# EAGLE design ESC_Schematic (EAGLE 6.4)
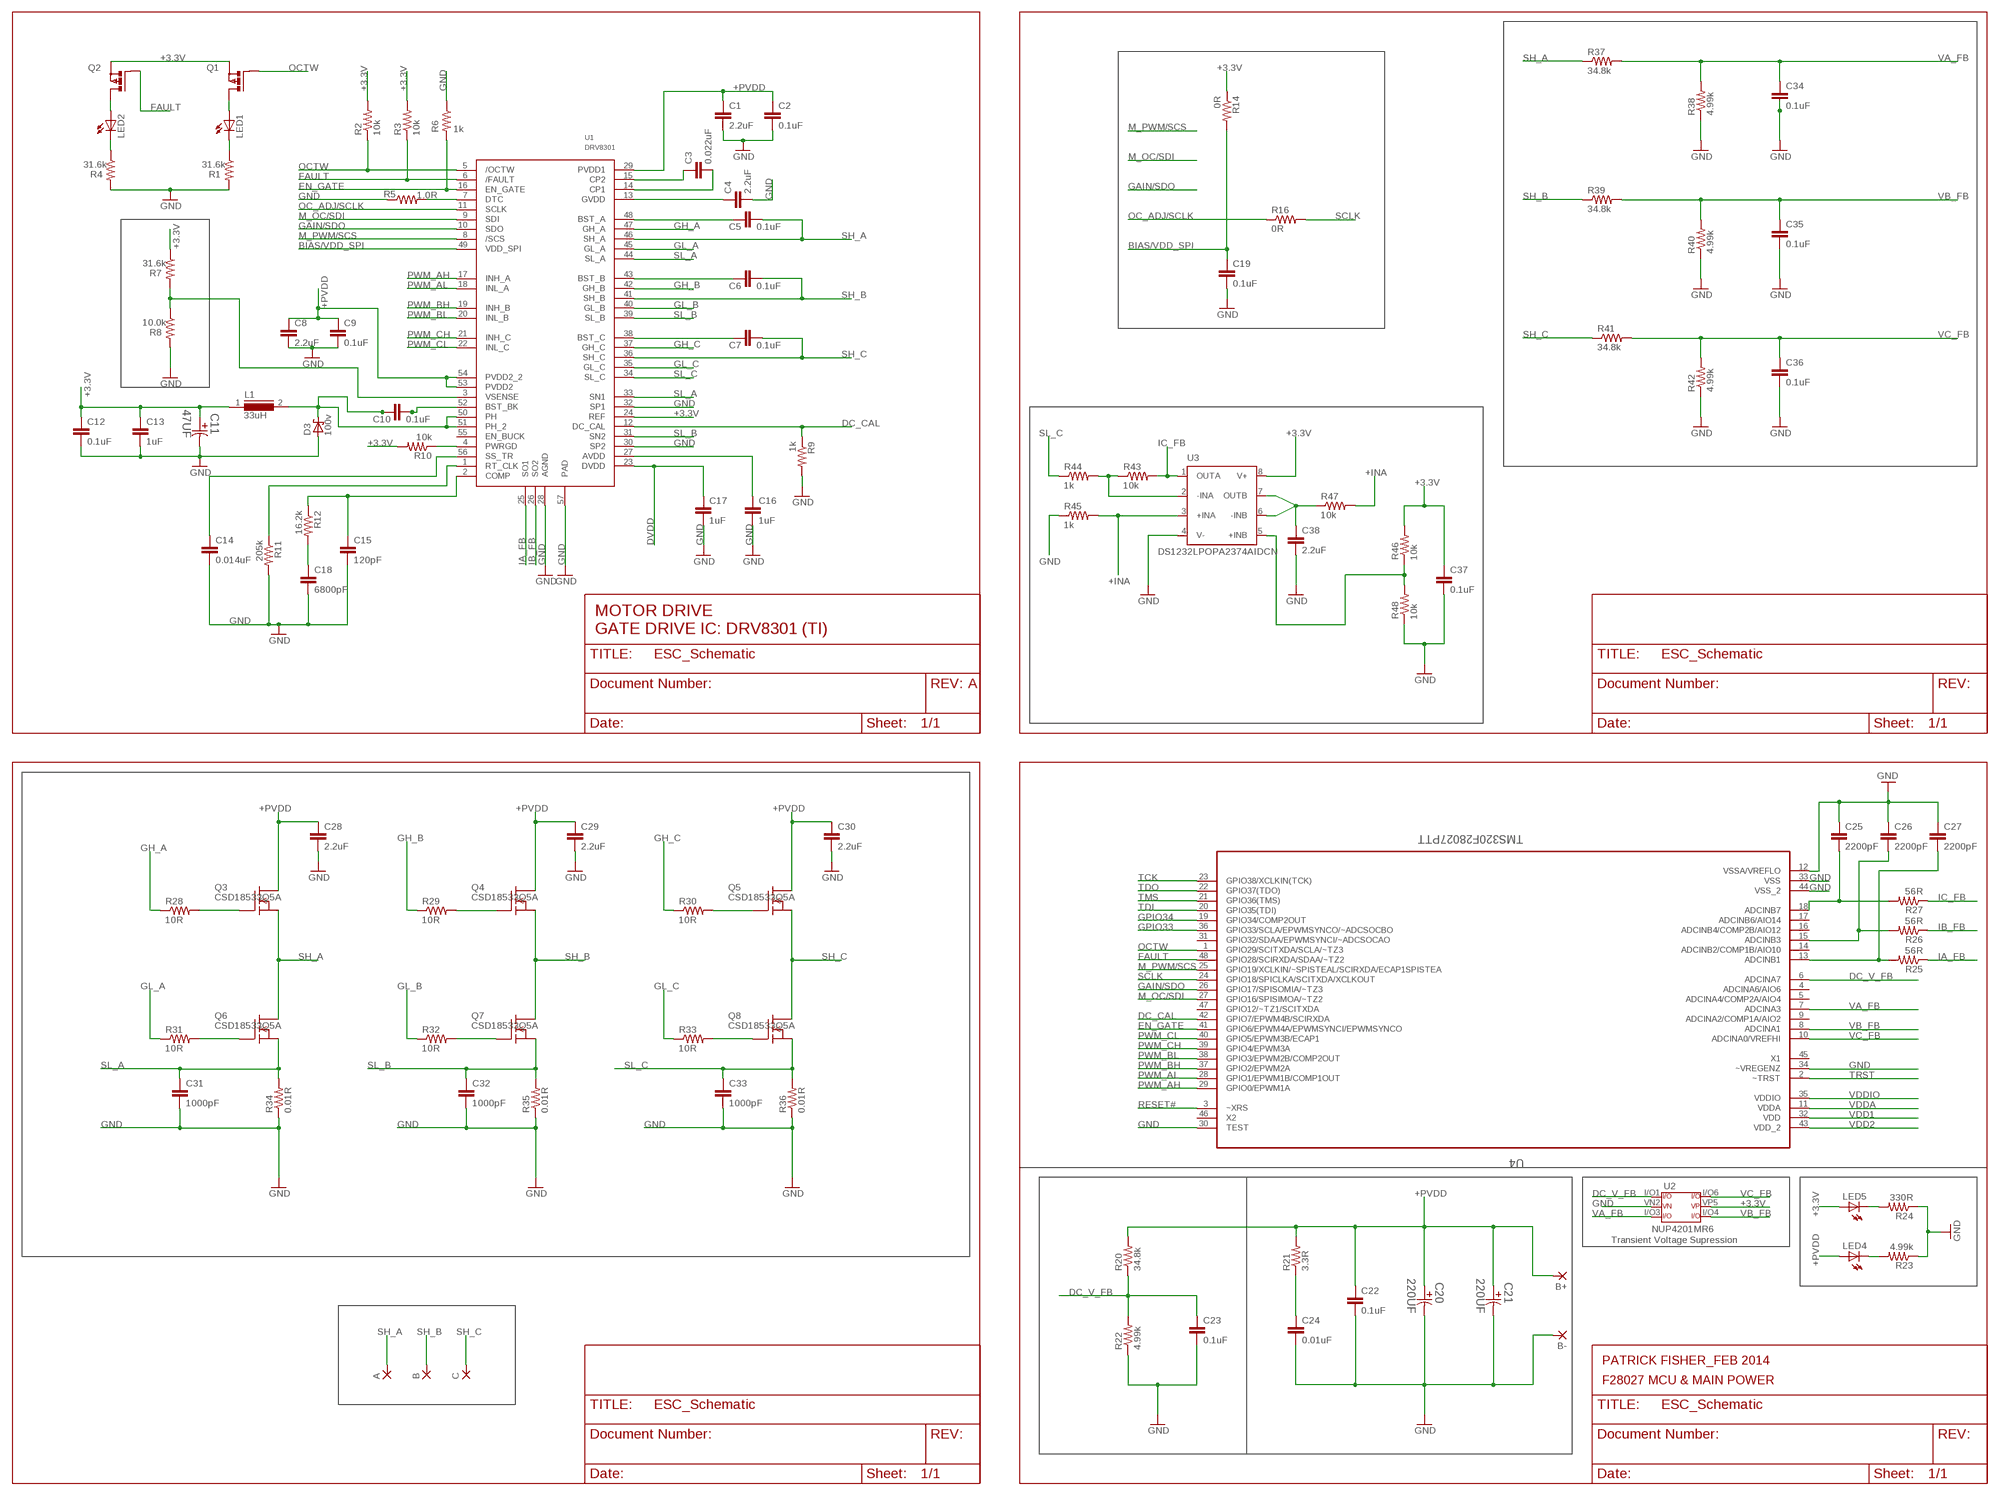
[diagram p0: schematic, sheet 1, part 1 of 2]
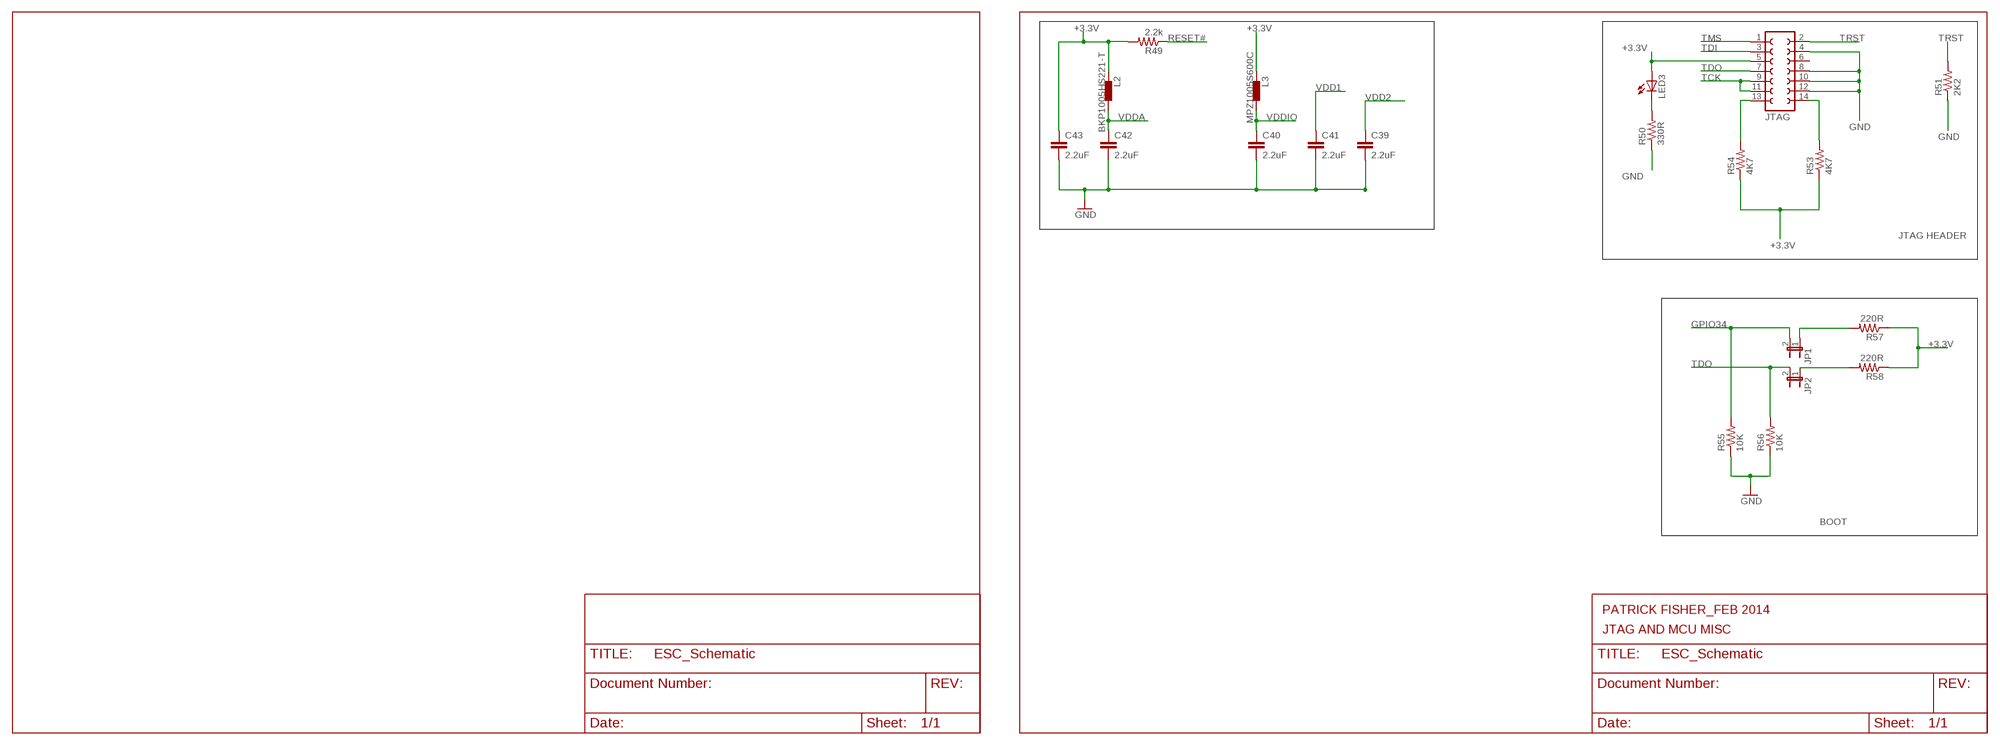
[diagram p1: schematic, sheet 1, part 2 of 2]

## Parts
A  WIREPAD4,16O1,6  [4,16O1,6]
B  WIREPAD4,16O1,6  [4,16O1,6]
B+  WIREPAD4,16O1,6  [4,16O1,6]
B-  WIREPAD4,16O1,6  [4,16O1,6]
C  WIREPAD4,16O1,6  [4,16O1,6]
C1  2.2uF  C-EUC1210  [C1210]
C2  0.1uF  C-EUC0603  [C0603]
C3  0.022uF  C-EUC0603  [C0603]
C4  2.2uF  C-EUC0805  [C0805]
C5  0.1uF  C-EUC0603  [C0603]
C6  0.1uF  C-EUC0603  [C0603]
C7  0.1uF  C-EUC0603  [C0603]
C8  2.2uF  C-EUC1210  [C1210]
C9  0.1uF  C-EUC0603  [C0603]
C10  0.1uF  C-EUC0603  [C0603]
C11  47UF  EEE-FK1E470P-CASE-D  [CAPAE660X610N]
C12  0.1uF  C-EUC0603  [C0603]
C13  1uF  C-EUC0603  [C0603]
C14  0.014uF  C-EUC0603  [C0603]
C15  120pF  C-EUC0603  [C0603]
C16  1uF  C-EUC0603  [C0603]
C17  1uF  C-EUC0603  [C0603]
C18  6800pF  C-EUC0603  [C0603]
C19  0.1uF  C-EUC0603  [C0603]
C20  220UF  EEE-FC1H221P-CASE-G  [CAPAE1030X1050N]
C21  220UF  EEE-FC1H221P-CASE-G  [CAPAE1030X1050N]
C22  0.1uF  C-EUC0603  [C0603]
C23  0.1uF  C-EUC0603  [C0603]
C24  0.01uF  C-EUC0603  [C0603]
C25  2200pF  C-EUC0603  [C0603]
C26  2200pF  C-EUC0603  [C0603]
C27  2200pF  C-EUC0603  [C0603]
C28  2.2uF  C-EUC1210  [C1210]
C29  2.2uF  C-EUC1210  [C1210]
C30  2.2uF  C-EUC1210  [C1210]
C31  1000pF  C-EUC0603  [C0603]
C32  1000pF  C-EUC0603  [C0603]
C33  1000pF  C-EUC0603  [C0603]
C34  0.1uF  C-EUC0603  [C0603]
C35  0.1uF  C-EUC0603  [C0603]
C36  0.1uF  C-EUC0603  [C0603]
C37  0.1uF  C-EUC0603  [C0603]
C38  2.2uF  C-EUC0603  [C0603]
C39  2.2uF  C-EUC0402K  [C0402K]
C40  2.2uF  C-EUC0402K  [C0402K]
C41  2.2uF  C-EUC0402K  [C0402K]
C42  2.2uF  C-EUC0402K  [C0402K]
C43  2.2uF  C-EUC0402K  [C0402K]
D3  100v  SCHOTTKY-DIODESMD  [SMB]
JP1  JP1E  [JP1]
JP2  JP1E  [JP1]
JTAG  FE07-2  [FE07-2]
L1  33uH  DR74  [DR74]
L2  220R  BLM15HB121SN1  [0402]
L3  60R  BLM15HB121SN1  [0402]
LED1  LEDCHIP-LED0805  [CHIP-LED0805]
LED2  LEDCHIP-LED0805  [CHIP-LED0805]
LED3  LEDCHIP-LED0805  [CHIP-LED0805]
LED4  LEDCHIP-LED0805  [CHIP-LED0805]
LED5  LEDCHIP-LED0805  [CHIP-LED0805]
Q1  P-MOSFET-SO8  [SOT23]
Q2  P-MOSFET-SO8  [SOT23]
Q3  CSD18533Q5A  [SON5*6]
Q4  CSD18533Q5A  [SON5*6]
Q5  CSD18533Q5A  [SON5*6]
Q6  CSD18533Q5A  [SON5*6]
Q7  CSD18533Q5A  [SON5*6]
Q8  CSD18533Q5A  [SON5*6]
R1  31.6k  R-US_R0603  [R0603]
R2  10k  R-US_R0603  [R0603]
R3  10k  R-US_R0603  [R0603]
R4  31.6k  R-US_R0603  [R0603]
R5  1.0R  R-US_R0603  [R0603]
R6  1k  R-US_R0603  [R0603]
R7  31.6k  R-US_R0603  [R0603]
R8  10.0k  R-US_R0603  [R0603]
R9  1k  R-US_R0603  [R0603]
R10  10k  R-US_R0603  [R0603]
R11  205k  R-US_R0603  [R0603]
R12  16.2k  R-US_R0603  [R0603]
R14  0R  R-US_R0603  [R0603]
R16  0R  R-US_R0603  [R0603]
R20  34.8k  R-US_R0603  [R0603]
R21  3.3R  R-US_R1206  [R1206]
R22  4.99k  R-US_R0603  [R0603]
R23  4.99k  R-US_R0603  [R0603]
R24  330R  R-US_R0603  [R0603]
R25  56R  R-US_R0603  [R0603]
R26  56R  R-US_R0603  [R0603]
R27  56R  R-US_R0603  [R0603]
R28  10R  R-US_R0603  [R0603]
R29  10R  R-US_R0603  [R0603]
R30  10R  R-US_R0603  [R0603]
R31  10R  R-US_R0603  [R0603]
R32  10R  R-US_R0603  [R0603]
R33  10R  R-US_R0603  [R0603]
R34  0.01R  R-US_R2512  [R2512]
R35  0.01R  R-US_R2512  [R2512]
R36  0.01R  R-US_R2512  [R2512]
R37  34.8k  R-US_R0603  [R0603]
R38  4.99k  R-US_R0603  [R0603]
R39  34.8k  R-US_R0603  [R0603]
R40  4.99k  R-US_R0603  [R0603]
R41  34.8k  R-US_R0603  [R0603]
R42  4.99k  R-US_R0603  [R0603]
R43  10k  R-US_R0603  [R0603]
R44  1k  R-US_R0603  [R0603]
R45  1k  R-US_R0603  [R0603]
R46  10k  R-US_R0603  [R0603]
R47  10k  R-US_R0603  [R0603]
R48  10k  R-US_R0603  [R0603]
R49  2.2k  R-US_R0402  [R0402]
R50  330R  R-US_R0603  [R0603]
R51  2K2  R-US_R0603  [R0603]
R53  4K7  R-US_R0603  [R0603]
R54  4K7  R-US_R0603  [R0603]
R55  10K  R-US_R0603  [R0603]
R56  10K  R-US_R0603  [R0603]
R57  220R  R-US_R0603  [R0603]
R58  220R  R-US_R0603  [R0603]
U1  DRV8301  [TSSOP56P]
U2  DIL6  [SOT23-6]
U3  DS1232LPOPA2374AIDCN  [DCN-R-PDSO-G8]
U4  TMS320F28027PTT  [QFP50P900X900X160-48N]

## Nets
+3.3V: C11.1 C12.1 C13.1 C37.1 C43.1 JTAG.5 L1.1 L2.1 L3.1 LED3.A LED5.A Q1.2(S) Q2.2(S) R2.2 R3.2 R7.1 R10.2 R14.1 R46.2 R49.2 R53.1 R54.1 R57.1 R58.1 U1.24(REF) U2.VP5 U3.8(V+)
+INA: R45.2 R47.2 U3.3(+INA)
+PVDD: B+.1(P) C1.1 C2.1 C8.1 C9.1 C20.1 C21.1 C22.1 C28.1 C29.1 C30.1 LED4.A Q3.5(D) Q3.6(D) Q3.7(D) Q3.8(D) Q3.9(D) Q4.5(D) Q4.6(D) Q4.7(D) Q4.8(D) Q4.9(D) Q5.5(D) Q5.6(D) Q5.7(D) Q5.8(D) Q5.9(D) R20.2 R21.2 U1.29(PVDD1) U1.53(PVDD2) U1.54(PVDD2_2)
BIAS/VDD_SPI: C19.1 R14.2 U1.49(VDD_SPI)
DC_CAL: R9.1 U1.12(DC_CAL) U4.42(GPIO7/EPWM4B/SCIRXDA)
DC_V_FB: C23.1 R20.1 R22.2 U2.I/O1 U4.6(ADCINA7)
DVDD: C17.1 U1.23(DVDD)
EN_GATE: R6.2 U1.16(EN_GATE) U4.41(GPIO6/EPWM4A/EPWMSYNCI/EPWMSYNCO)
FAULT: Q2.1(G) R3.1 U1.6(/FAULT) U4.48(GPIO28/SCIRXDA/SDAA/~TZ2)
GAIN/SDO: U1.10(SDO) U4.26(GPIO17/SPISOMIA/~TZ3)
GH_A: R28.1 U1.47(GH_A)
GH_B: R29.1 U1.42(GH_B)
GH_C: R30.1 U1.37(GH_C)
GL_A: R31.1 U1.45(GL_A)
GL_B: R32.1 U1.40(GL_B)
GL_C: R33.1 U1.35(GL_C)
GND: B-.1(P) C1.2 C2.2 C4.2 C8.2 C9.2 C11.2 C12.2 C13.2 C14.2 C15.2 C16.2 C17.2 C18.2 C19.2 C20.2 C21.2 C22.2 C23.2 C24.2 C25.1 C26.1 C27.1 C28.2 C29.2 C30.2 C31.2 C32.2 C33.2 C34.2 C35.2 C36.2 C37.2 C38.2 C39.2 C40.2 C41.2 C42.2 C43.2 D3.A JTAG.4 JTAG.8 JTAG.10 JTAG.12 R1.2 R4.2 R5.1 R6.1 R8.2 R9.2 R11.2 R22.1 R23.1 R24.1 R34.1 R35.1 R36.1 R38.1 R40.1 R42.1 R45.1 R48.1 R50.1 R51.1 R55.1 R56.1 U1.28(AGND) U1.30(SP2) U1.32(SP1) U1.57(PAD) U2.VN2 U3.4(V-) U4.12(VSSA/VREFLO) U4.30(TEST) U4.33(VSS) U4.34(~VREGENZ) U4.44(VSS_2)
GPIO33: U4.36(GPIO33/SCLA/EPWMSYNCO/~ADCSOCBO)
GPIO34: JP1.2 R55.2 U4.19(GPIO34/COMP2OUT)
IA_FB: R25.1 U1.25(SO1)
IB_FB: R26.1 U1.26(SO2)
IC_FB: R27.1 R43.2 U3.1(OUTA)
M_OC/SDI: U1.9(SDI) U4.27(GPIO16/SPISIMOA/~TZ2)
M_PWM/SCS: U1.8(/SCS) U4.25(GPIO19/XCLKIN/~SPISTEAL/SCIRXDA/ECAP1SPISTEA)
N$1: R10.1 U1.4(PWRGD)
N$2: R7.2 R8.1 U1.3(VSENSE)
N$3: C10.2 U1.52(BST_BK)
N$4: R5.2 U1.7(DTC)
N$5: C10.1 D3.C L1.2 U1.50(PH) U1.51(PH_2)
N$6: C18.1 R12.2
N$7: C14.1 U1.56(SS_TR)
N$8: LED1.A Q1.3(D)
N$9: C15.1 R12.1 U1.2(COMP)
N$10: C3.1 U1.15(CP2)
N$11: R11.1 U1.1(RT_CLK)
N$12: C3.2 U1.14(CP1)
N$13: C4.1 U1.13(GVDD)
N$14: C6.1 U1.43(BST_B)
N$15: C5.1 U1.48(BST_A)
N$16: C7.1 U1.38(BST_C)
N$17: LED1.C R1.1
N$18: LED2.A Q2.3(D)
N$19: LED2.C R4.1
N$21: C38.1 R47.1 U3.6(-INB) U3.7(OUTB)
N$22: R46.1 R48.2 U3.5(+INB)
N$23: C16.1 U1.27(AVDD)
N$24: Q3.4(G) R28.2
N$25: Q4.4(G) R29.2
N$26: R43.1 R44.2 U3.2(-INA)
N$27: Q5.4(G) R30.2
N$28: Q7.4(G) R32.2
N$29: Q8.4(G) R33.2
N$30: Q6.4(G) R31.2
N$31: C26.2 R26.2 U4.15(ADCINB3)
N$32: C27.2 R25.2 U4.13(ADCINB1)
N$33: LED3.C R50.2
N$34: LED4.C R23.2
N$35: C25.2 R27.2 U4.18(ADCINB7)
N$36: LED5.C R24.2
N$39: JTAG.13 R54.2
N$40: JTAG.14 R53.2
N$42: JP1.1 R57.2
N$44: C24.1 R21.1
N$45: JP2.1 R58.2
OC_ADJ/SCLK: R16.1 U1.11(SCLK)
OCTW: Q1.1(G) R2.1 U1.5(/OCTW) U4.1(GPIO29/SCITXDA/SCLA/~TZ3)
PWM_AH: U1.17(INH_A) U4.29(GPIO0/EPWM1A)
PWM_AL: U1.18(INL_A) U4.28(GPIO1/EPWM1B/COMP1OUT)
PWM_BH: U1.19(INH_B) U4.37(GPIO2/EPWM2A)
PWM_BL: U1.20(INL_B) U4.38(GPIO3/EPWM2B/COMP2OUT)
PWM_CH: U1.21(INH_C) U4.39(GPIO4/EPWM3A)
PWM_CL: U1.22(INL_C) U4.40(GPIO5/EPWM3B/ECAP1)
RESET#: R49.1 U4.3(~XRS)
SCLK: R16.2 U4.24(GPIO18/SPICLKA/SCITXDA/XCLKOUT)
SH_A: A.1(P) C5.2 Q3.1(S) Q3.2(S) Q3.3(S) Q6.5(D) Q6.6(D) Q6.7(D) Q6.8(D) Q6.9(D) R37.1 U1.46(SH_A)
SH_B: B.1(P) C6.2 Q4.1(S) Q4.2(S) Q4.3(S) Q7.5(D) Q7.6(D) Q7.7(D) Q7.8(D) Q7.9(D) R39.1 U1.41(SH_B)
SH_C: C7.2 C.1(P) Q5.1(S) Q5.2(S) Q5.3(S) Q8.5(D) Q8.6(D) Q8.7(D) Q8.8(D) Q8.9(D) R41.1 U1.36(SH_C)
SL_A: C31.1 Q6.1(S) Q6.2(S) Q6.3(S) R34.2 U1.33(SN1) U1.44(SL_A)
SL_B: C32.1 Q7.1(S) Q7.2(S) Q7.3(S) R35.2 U1.31(SN2) U1.39(SL_B)
SL_C: C33.1 Q8.1(S) Q8.2(S) Q8.3(S) R36.2 R44.1 U1.34(SL_C)
TCK: JTAG.9 JTAG.11 U4.23(GPIO38/XCLKIN(TCK))
TDI: JTAG.3 U4.20(GPIO35(TDI))
TDO: JP2.2 JTAG.7 R56.2 U4.22(GPIO37(TDO))
TMS: JTAG.1 U4.21(GPIO36(TMS))
TRST: JTAG.2 R51.2 U4.2(~TRST)
VA_FB: C34.1 R37.2 R38.2 U2.I/O3 U4.7(ADCINA3)
VB_FB: C35.1 R39.2 R40.2 U2.I/O4 U4.8(ADCINA1)
VC_FB: C36.1 R41.2 R42.2 U2.I/O6 U4.10(ADCINA0/VREFHI)
VDD1: C41.1 U4.32(VDD)
VDD2: C39.1 U4.43(VDD_2)
VDDA: C42.1 L2.2 U4.11(VDDA)
VDDIO: C40.1 L3.2 U4.35(VDDIO)
Unconnected: JTAG.6 U1.55(EN_BUCK) U4.4(ADCINA6/AIO6) U4.5(ADCINA4/COMP2A/AIO4) U4.9(ADCINA2/COMP1A/AIO2) U4.14(ADCINB2/COMP1B/AIO10) U4.16(ADCINB4/COMP2B/AIO12) U4.17(ADCINB6/AIO14) U4.31(GPIO32/SDAA/EPWMSYNCI/~ADCSOCAO) U4.45(X1) U4.46(X2) U4.47(GPIO12/~TZ1/SCITXDA)

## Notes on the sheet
- MOTOR DRIVE
  GATE DRIVE IC: DRV8301 (TI)
- A
- NUP4201MR6
- Transient Voltage Supression
- PATRICK FISHER_FEB 2014
- F28027 MCU & MAIN POWER
- BKP1005HS221-T | MPZ1005S600C
- JTAG HEADER
- BOOT
- PATRICK FISHER_FEB 2014
- JTAG AND MCU MISC

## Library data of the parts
A B B+ B- C = wirepad:WIREPAD: Wire PAD connect wire on PCB
C1-C10 C12-C19 C22-C43 = rcl:C-EU: CAPACITOR, European symbol
C11 = Panasonic-EEEFK_EEEFP:EEE-: Aluminum Electrolytic Capacitors,Surface Mount Type; MPN: EEE-FK1E470P; OC_FARNELL: 9695753; OC_NEWARK: 87K0936; PACKAGE: CASE-D; SUPPLIER: PANASONIC; TOLERANCE: ±20 %; VOLTAGERATING: 25V
C20 C21 = Panasonic-EEE0_EEE1_EEE2_EEEFC:EEE-: Aluminum Electrolytic Capacitors,Surface Mount Type; MPN: EEE-FC1H221P; OC_FARNELL: 2284641; OC_NEWARK: 53W3650; PACKAGE: CASE-G; SUPPLIER: PANASONIC; TOLERANCE: 20%; VOLTAGERATING: 50V
D3 = diode:SCHOTTKY-DIODE: Schottky Diode
JP1 JP2 = jumper:JP1E: JUMPER
JTAG = con-lsta:FE07-2: FEMALE HEADER; OC_FARNELL: unknown; OC_NEWARK: unknown
L1 = inductors:DR74: High Power Density, High Efficiency, Shielded Inductors
L2 L3 = inductors:BLM15H: EMIFIL (R) Chip Ferrite Bead for GHz Noise
LED1-LED5 = led:LED: LED
Q1 Q2 = FET SOT23(good):P-MOSFET-SO8: P-Channel MOSFET Example: FDS4435A; P-Channel Logic Level PowerTrench® MOSFET FDS4465; P-Channel 1.8V Specified PowerTrench® MOSFET Source: www.fairchildsemi.com
Q3-Q8 = CSD18533Q5A:CSD18533Q5A: 60V N-Channel PowerTrench TM MOSFET FAIRCHILD FDS5680.pdf
R1-R12 R14 R16 R20-R51 R53-R58 = resistor:R-US_: RESISTOR, American symbol
U1 = sc_usercreated:DRV8301
U2 = NUP4201MR6:DIL6: Dual In Line / Socket
U3 = OPA2374AIDCN:DS1232LP: Low Power MicroMonitor Chip Source: DALLAS SEMICONDUCTOR .. 1232lp.pdf
U4 = F28027F:TMS320F28027PTT: Piccolo Microcontrollers; MPN: TMS320F28027PTT; OC_FARNELL: 2113746; OC_NEWARK: 50R8075; PACKAGE: PQFP-48; SUPPLIER: Texas Instruments

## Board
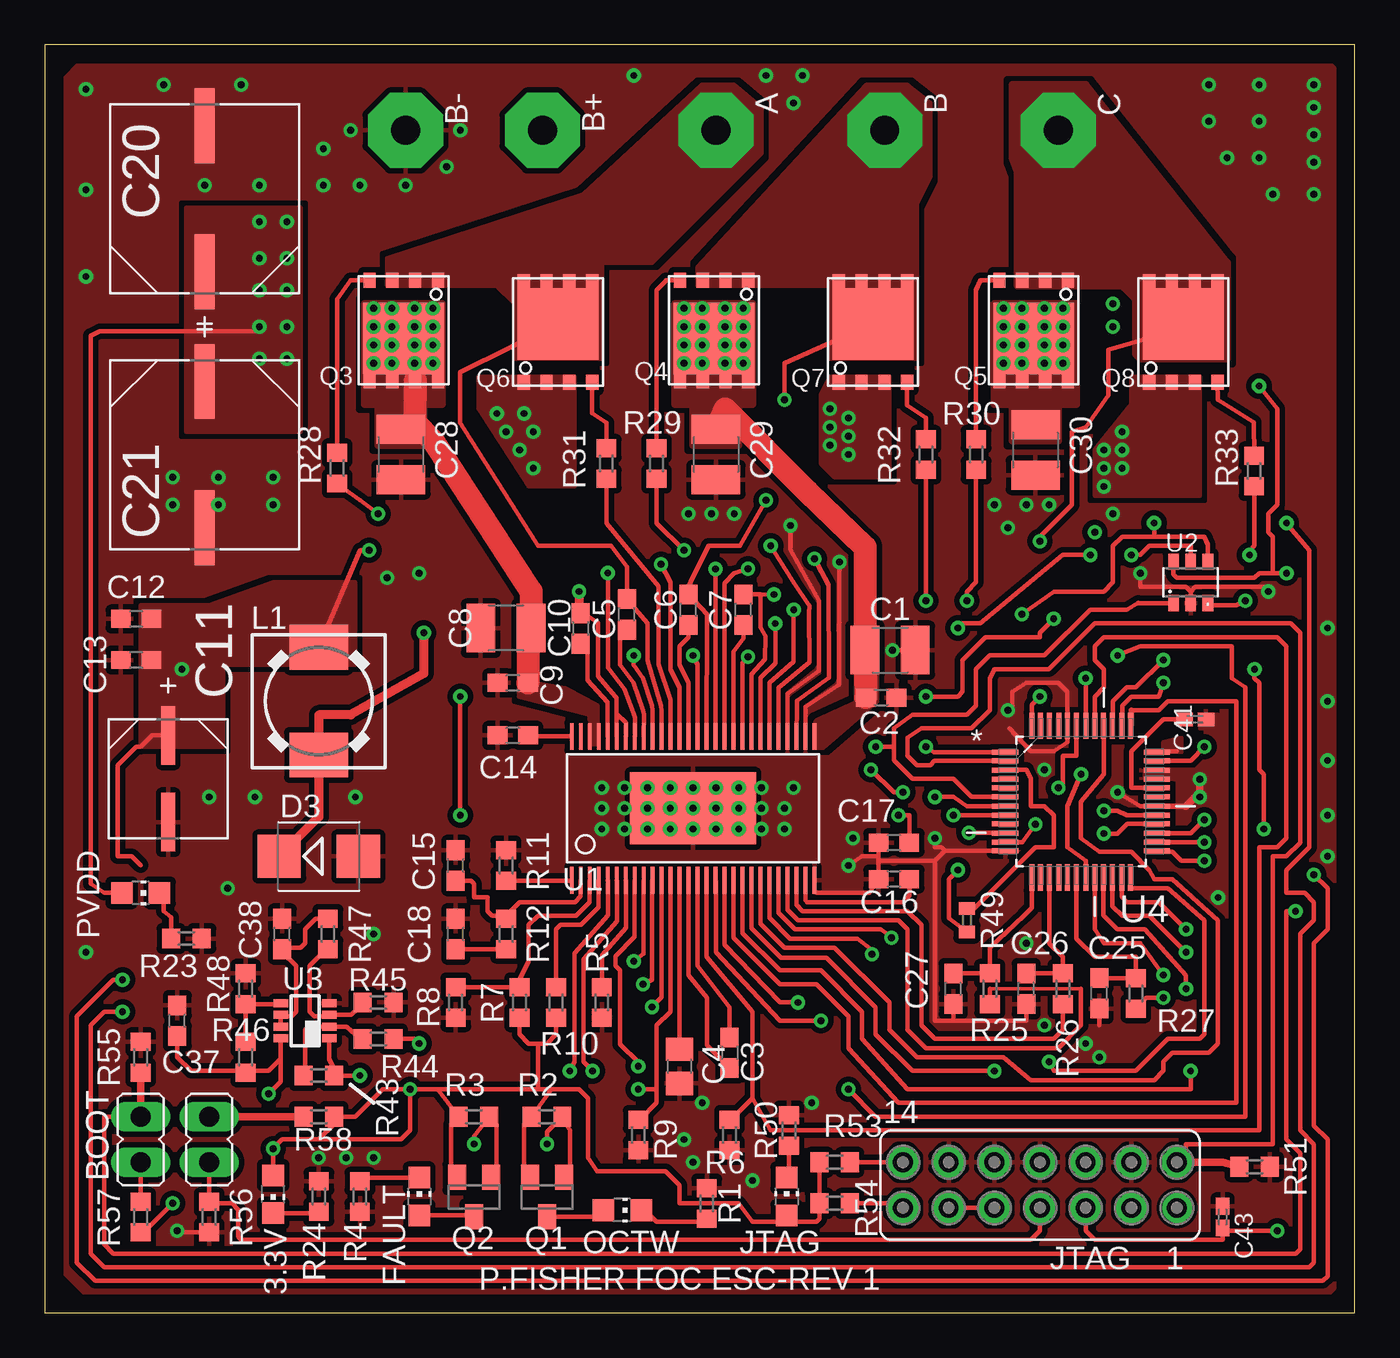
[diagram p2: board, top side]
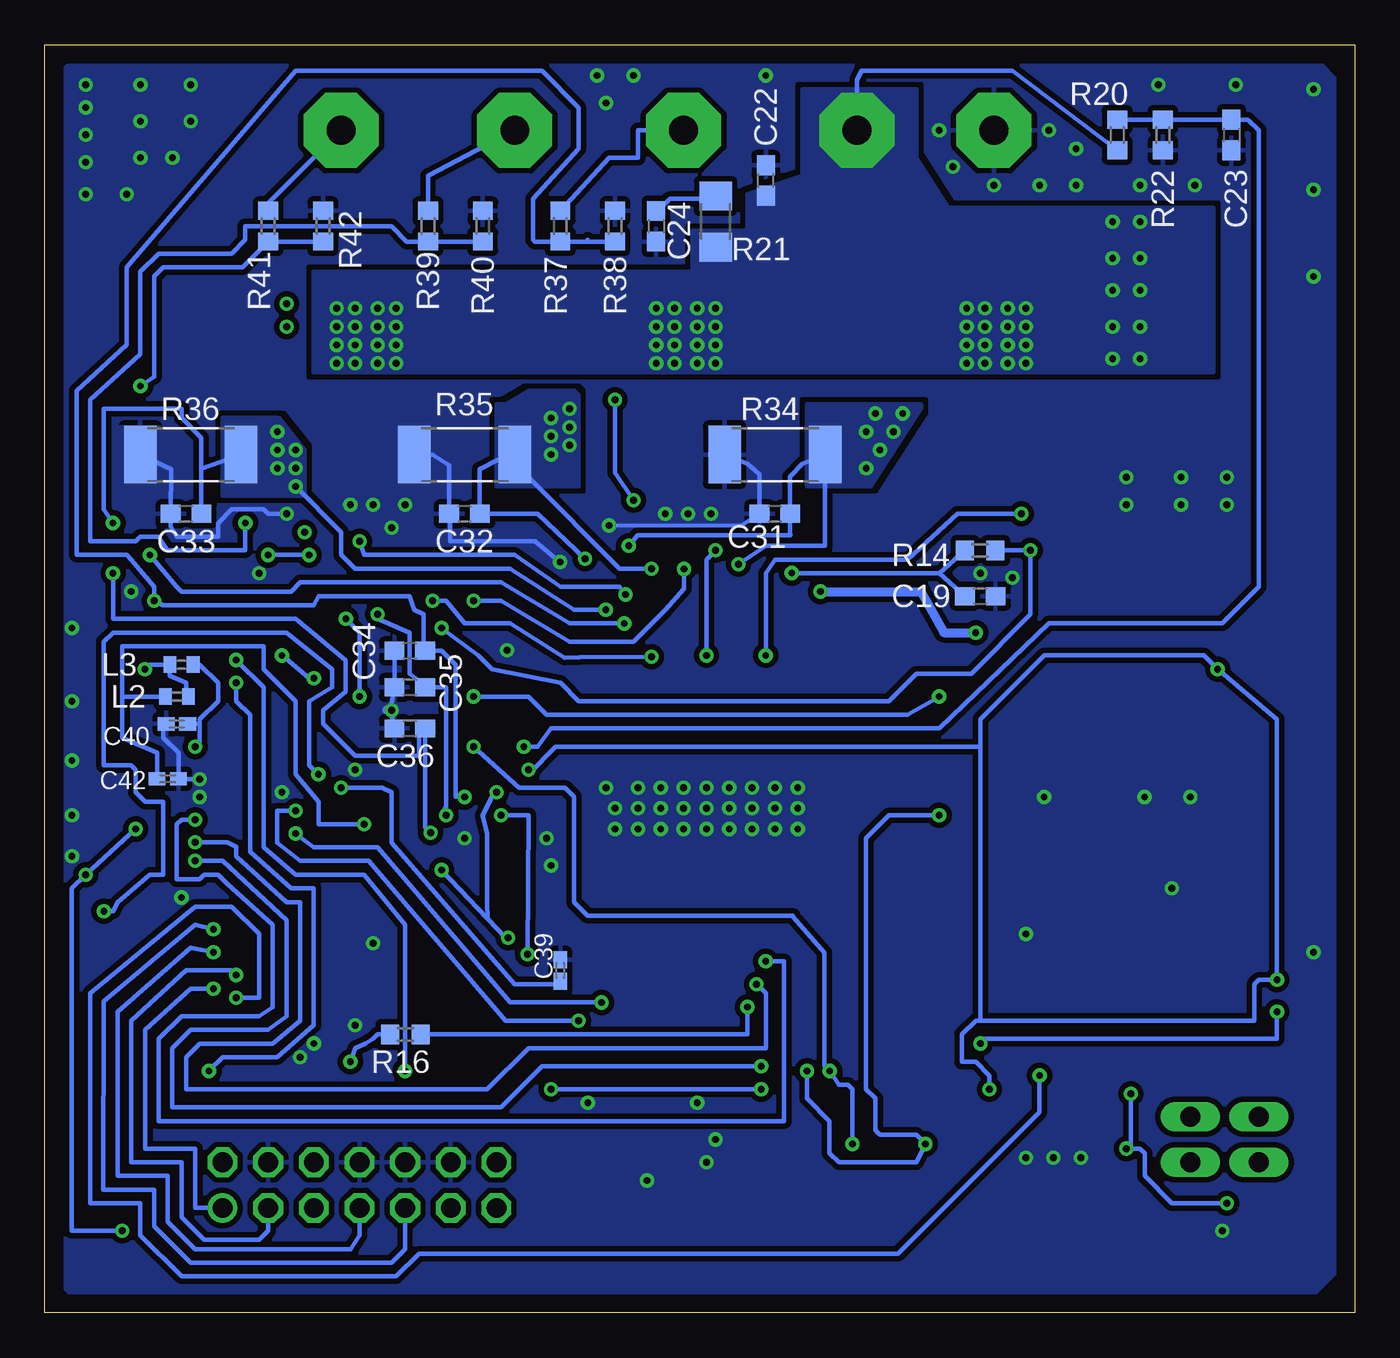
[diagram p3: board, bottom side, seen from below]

Size 72.88 x 70.54 mm. Coordinates in mm from the lower left corner, seen from the top.
Outline: 0,0 72.88,0 72.88,70.54 0,70.54 0,0
Copper layers (1*16): Top 0.035mm / dielectric 1.5mm / Bottom 0.035mm
Design rules "default *": minimum track width 5mil, minimum drill 15mil, track to track 8mil, track to pad 6mil, pad to pad 6mil, via to via 10mil, smd to smd 6mil, copper to edge 40mil, drill to drill 8mil, minimum pad ring 10mil, minimum via ring 8mil, stop-mask expansion 4mil, vias tented up to drill 0mil, thermal gap 12mil

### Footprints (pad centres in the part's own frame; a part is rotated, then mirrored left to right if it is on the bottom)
4,16O1,6 = drill 1.6 pad 4.166 octagon: 1 0,0
C1210 = smd 1.6 x 2.7: 1 -1.4,0; 2 1.4,0
C0603 = smd 1.1 x 1: 1 -0.85,0; 2 0.85,0
C0805 = smd 1.3 x 1.5: 1 -0.95,0; 2 0.95,0
CAPAE660X610N = smd 3.251 x 0.762: 1 -2.413,0; 2 2.413,0
CAPAE1030X1050N = smd 4.166 x 1.092: 1 -4.064,0; 2 4.064,0
C0402K = smd 0.925 x 0.74: 1 -0.6,0; 2 0.6,0
SMB = smd 2.4 x 2.4: A 2.2,0; C -2.2,0
JP1 = drill 1.1 long: 1 0,-1.27; 2 0,1.27
FE07-2 = drill 1.1: 1 -7.62,1.27 | drill 1.1 octagon: 2 -7.62,-1.27; 3 -5.08,1.27; 4 -5.08,-1.27; 5 -2.54,1.27; 6 -2.54,-1.27; 7 0,1.27; 8 0,-1.27; 9 2.54,1.27; 10 2.54,-1.27; 11 5.08,1.27; 12 5.08,-1.27; 13 7.62,1.27; 14 7.62,-1.27
DR74 = smd 2.5 x 3.25: 1 -3,0; 2 3,0
0402 = smd 0.7 x 0.9: 1 -0.65,0; 2 0.65,0
CHIP-LED0805 = smd 1.2 x 1.2: A 0,-1.05; C 0,1.05
SOT23 = smd 1 x 1.4: 1 -0.95,-1.2; 2 0.95,-1.2; 3 0,1
SON5*6 = smd 0.85 x 0.68: 1 -3.095,1.805; 2 -3.095,0.535; 3 -3.095,-0.735; 4 -3.095,-2.005; 5 2.495,-2.005; 6 2.495,-0.735; 7 2.495,0.535; 8 2.495,1.805 | smd 4 x 4.5: 9 0.15,-0.1
R0603 = smd 1 x 1.1: 1 -0.85,0; 2 0.85,0
R1206 = smd 1.6 x 1.803: 1 -1.422,0; 2 1.422,0
R2512 = smd 1.8 x 3.2: 1 -2.8,0; 2 2.8,0
R0402 = smd 0.7 x 0.9: 1 -0.65,0; 2 0.65,0
TSSOP56P = smd 1.5 x 0.21: 1 -4,6.75; 2 -4,6.25; 3 -4,5.75; 4 -4,5.25; 5 -4,4.75; 6 -4,4.25; 7 -4,3.75; 8 -4,3.25; 9 -4,2.75; 10 -4,2.25; 11 -4,1.75; 12 -4,1.25; 13 -4,0.75; 14 -4,0.25; 15 -4,-0.25; 16 -4,-0.75; 17 -4,-1.25; 18 -4,-1.75; 19 -4,-2.25; 20 -4,-2.75; 21 -4,-3.25; 22 -4,-3.75; 23 -4,-4.25; 24 -4,-4.75; 25 -4,-5.25; 26 -4,-5.75; 27 -4,-6.25; 28 -4,-6.75; 29 4,-6.75; 30 4,-6.25; 31 4,-5.75; 32 4,-5.25; 33 4,-4.75; 34 4,-4.25; 35 4,-3.75; 36 4,-3.25; 37 4,-2.75; 38 4,-2.25; 39 4,-1.75; 40 4,-1.25; 41 4,-0.75; 42 4,-0.25; 43 4,0.25; 44 4,0.75; 45 4,1.25; 46 4,1.75; 47 4,2.25; 48 4,2.75; 49 4,3.25; 50 4,3.75; 51 4,4.25; 52 4,4.75; 53 4,5.25; 54 4,5.75; 55 4,6.25; 56 4,6.75 | smd 4 x 7: 57 0,0
SOT23-6 = smd 0.6 x 0.9: I/O1 -0.95,-1.15; I/O3 0.95,-1.15; I/O4 0.95,1.15; I/O6 -0.95,1.15; VN2 0,-1.15; VP5 0,1.15
DCN-R-PDSO-G8 = smd 0.45 x 0.8: 1 -0.975,-1.35; 2 -0.325,-1.35; 3 0.325,-1.35; 4 0.975,-1.35; 5 0.975,1.35; 6 0.325,1.35; 7 -0.325,1.35; 8 -0.975,1.35
QFP50P900X900X160-48N = smd 1.473 x 0.279: 1 -4.216,2.743; 2 -4.216,2.261; 3 -4.216,1.753; 4 -4.216,1.245; 5 -4.216,0.762; 6 -4.216,0.254; 7 -4.216,-0.254; 8 -4.216,-0.762; 9 -4.216,-1.245; 10 -4.216,-1.753; 11 -4.216,-2.261; 12 -4.216,-2.743; 25 4.216,-2.743; 26 4.216,-2.261; 27 4.216,-1.753; 28 4.216,-1.245; 29 4.216,-0.762; 30 4.216,-0.254; 31 4.216,0.254; 32 4.216,0.762; 33 4.216,1.245; 34 4.216,1.753; 35 4.216,2.261; 36 4.216,2.743 | smd 0.279 x 1.473: 13 -2.743,-4.216; 14 -2.261,-4.216; 15 -1.753,-4.216; 16 -1.245,-4.216; 17 -0.762,-4.216; 18 -0.254,-4.216; 19 0.254,-4.216; 20 0.762,-4.216; 21 1.245,-4.216; 22 1.753,-4.216; 23 2.261,-4.216; 24 2.743,-4.216; 37 2.743,4.216; 38 2.261,4.216; 39 1.753,4.216; 40 1.245,4.216; 41 0.762,4.216; 42 0.254,4.216; 43 -0.254,4.216; 44 -0.762,4.216; 45 -1.245,4.216; 46 -1.753,4.216; 47 -2.261,4.216; 48 -2.743,4.216

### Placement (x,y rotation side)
A  37.34,65.79 270 top
B  46.74,65.79 270 top
B+  27.69,65.79 270 top
B-  20.07,65.79 270 top
C  56.39,65.79 270 top
C1  47.03,36.87 0 top
C2  46.53,34.23 0 top
C3  38.1,14.48 270 top
C4  35.31,13.72 270 top
C5  32.39,38.86 90 top
C6  35.81,39.12 90 top
C7  38.86,39.12 90 top
C8  25.65,38.1 180 top
C9  26.04,35.05 180 top
C10  29.79,38.07 270 top
C11  6.86,29.72 270 top
C12  5.08,38.61 180 top
C13  5.08,36.32 180 top
C14  26.04,32.13 180 top
C15  22.86,24.89 90 top
C16  47.24,24.13 180 top
C17  47.24,26.16 180 top
C18  22.86,21.08 90 top
C19  20.83,39.88 0 bottom
C20  8.89,61.98 90 top
C21  8.89,47.75 270 top
C22  32.77,62.99 90 bottom
C23  6.86,65.53 270 bottom
C24  38.86,60.45 270 bottom
C25  58.67,17.78 90 top
C26  54.61,18.03 90 top
C27  50.55,18.03 90 top
C28  19.81,47.75 270 top
C29  37.34,47.75 270 top
C30  55.12,48.01 270 top
C31  32.26,44.45 180 bottom
C32  49.53,44.45 180 bottom
C33  65.02,44.45 180 bottom
C34  52.58,36.83 180 bottom
C35  52.58,34.8 180 bottom
C36  52.58,32.51 180 bottom
C37  7.37,16.26 90 top
C38  13.21,21.08 90 top
C39  44.2,19.05 90 bottom
C40  65.53,32.77 180 bottom
C41  64.01,33.02 0 top
C42  66.04,29.72 0 bottom
C43  65.53,5.33 90 top
D3  15.24,25.4 0 top
JP1  5.33,9.65 0 top
JP2  9.14,9.65 180 top
JTAG  55.37,7.11 180 top
L1  15.24,34.04 270 top
L2  65.53,34.29 180 bottom
L3  65.28,36.07 0 bottom
LED1  32.13,5.71 270 top
LED2  20.83,6.48 0 top
LED3  41.27,6.48 0 top
LED4  5.33,23.37 270 top
LED5  12.7,6.6 180 top
Q1  27.94,6.35 180 top
Q2  23.88,6.35 180 top
Q3  20.07,54.36 270 top
Q4  37.34,54.36 270 top
Q5  55.12,54.36 270 top
Q6  28.45,54.86 90 top
Q7  45.97,54.86 90 top
Q8  63.25,54.86 90 top
R1  36.83,6.1 90 top
R2  27.94,10.92 180 top
R3  23.88,10.92 180 top
R4  17.53,6.48 270 top
R5  30.99,17.27 90 top
R6  38.1,9.91 90 top
R7  26.42,17.27 90 top
R8  22.86,17.27 270 top
R9  33.02,9.91 270 top
R10  28.45,17.27 270 top
R11  25.65,24.89 90 top
R12  25.65,21.08 270 top
R14  20.83,42.42 180 bottom
R16  52.83,15.49 180 bottom
R20  13.21,65.53 270 bottom
R21  35.56,60.71 270 bottom
R22  10.67,65.53 90 bottom
R23  7.87,20.83 180 top
R24  15.24,6.48 270 top
R25  52.58,18.03 90 top
R26  56.64,18.03 90 top
R27  60.71,17.78 90 top
R28  16.26,46.99 90 top
R29  34.04,47.24 90 top
R30  51.82,47.75 90 top
R31  31.24,47.24 90 top
R32  49.02,47.75 90 top
R33  67.29,46.83 90 top
R34  32.26,47.75 0 bottom
R35  49.53,47.75 0 bottom
R36  64.77,47.75 0 bottom
R37  44.2,60.45 270 bottom
R38  41.15,60.45 270 bottom
R39  51.56,60.45 270 bottom
R40  48.51,60.45 270 bottom
R41  60.45,60.45 270 bottom
R42  57.4,60.45 270 bottom
R43  15.24,13.21 0 top
R44  18.54,15.24 180 top
R45  18.54,17.27 180 top
R46  11.18,14.22 270 top
R47  15.75,21.08 270 top
R48  11.18,18.03 270 top
R49  51.31,21.84 270 top
R50  41.4,10.16 270 top
R51  67.31,8.13 180 top
R53  43.94,8.38 0 top
R54  43.94,6.1 0 top
R55  5.33,14.22 270 top
R56  9.14,5.33 90 top
R57  5.33,5.33 90 top
R58  15.24,10.92 180 top
U1  36.07,28.07 90 top
U2  63.75,40.64 0 top
U3  14.48,16.26 90 top
U4  57.66,28.45 0 top

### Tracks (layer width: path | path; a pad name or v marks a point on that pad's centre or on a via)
+3.3V  (via drill 0.38 pad 0.64)
  Top 0.254: v18.03,42.42 17.53,42.42 L1.1 | 13.13,14.14 12.45,13.46 11.26,13.46 R46.2 11.09,13.46 8.13,13.46 7.37,14.22 C37.1 | 13.13,14.14 U3.8 | U1.24 40.82,22.44 40.82,22.26 41.74,21.34 46.48,21.34 47.1,20.95 47.1,20.94 v47.1,20.87 | 21.84,12.45 R3.2 22.61,10.5 22.61,7.62 Q2.2 | 21.84,12.45 27.43,12.45 | 27.43,12.45 28.19,12.45 | 28.19,12.45 29.72,12.45 30.23,11.94 30.23,8.64 30.73,7.87 34.54,7.87 35.31,7.11 35.31,6.1 38.61,6.1 39.37,5.08 41.12,5.08 LED3.A 41.37,5.08 42.93,5.08 43.09,5.25 R54.1 R53.1 | 28.19,12.45 R2.2 26.67,10.5 26.67,7.87 Q1.2 | R10.2 28.45,15.49 27.94,14.99 27.43,14.99 | 27.43,14.99 26.92,14.99 26.42,15.49 R7.1 | 27.43,14.99 27.43,12.45 | v20.32,12.45 18.8,12.45 17.27,10.92 R58.1 16.09,10.5 15.24,9.65 | v20.32,12.45 21.84,12.45 | JTAG.5 57.91,4.57 58.42,4.06 65.53,4.06 C43.1 65.69,4.57 v68.58,4.57 | v50.8,24.64 50.29,24.13 50.29,21.96 R49.2 | v60.45,42.16 60.96,42.16 61.47,42.67 63.75,42.67 U2.VP5 | R57.1 5.5,4.48 v7.11,6.1 | LED5.A v12.7,9.14 13.21,9.65 15.24,9.65 | 15.24,9.65 19.81,9.65 20.32,10.16 v20.32,12.45 | 13.13,14.14 13.13,12.87 v12.45,12.19 | C11.1 5.97,32.13 5.33,31.5 5.08,31.5 4.06,30.48 4.06,25.4 4.83,25.4 5.33,24.89 | v50.8,38.1 51.05,38.35 52.07,38.35 56.64,42.16 v58.17,42.16 | v67.31,35.81 67.31,35.31 67.56,35.05 67.56,30.23 67.82,29.97 v67.82,26.92 | v70.61,24.38 71.37,23.62 71.37,21.34 70.61,20.57 70.61,10.41 71.37,9.65 71.37,2.03 71.12,1.78 2.79,1.78 1.78,2.79 1.78,16.51 3.81,18.54 v4.32,18.54 | v45.97,30.23 47.24,28.96 v47.75,28.96
  Bottom 0.254: R14.1 v18.03,42.42 18.03,38.86 21.34,35.56 24.38,35.56 25.91,34.04 43.18,34.04 44.2,35.05 48.01,35.81 48.77,36.58 v50.8,38.1 | L2.1 65.02,34.43 65.02,35.05 65.93,35.45 L3.1 67.06,36.07 v67.31,35.81 | v7.11,6.1 10.16,6.1 11.68,7.62 11.68,8.89 11.94,9.14 12.45,9.14 | v12.45,12.19 12.45,9.14 | 12.45,9.14 v12.7,9.14 | v58.17,42.16 v60.45,42.16 | v67.82,26.92 v70.61,24.38 71.37,23.62 71.37,4.57 v68.58,4.57 | 20.83,16.26 5.59,16.26 5.59,18.29 5.33,18.54 v4.32,18.54 4.32,33.02 v7.62,35.81 8.38,36.58 17.27,36.58 20.83,33.02 20.83,31.5 | 20.83,16.26 21.08,16.26 21.84,15.49 21.84,13.97 21.08,13.97 20.32,13.21 v20.32,12.45 | 20.83,16.26 20.83,31.5 | 20.83,31.5 44.45,31.5 45.97,29.97 v45.97,30.23 | v47.75,28.96 48.01,28.7 48.51,27.69 48.26,26.67 48.26,22.86 48.23,21.93 47.24,20.87 | v47.1,20.87 47.24,20.87 | 47.24,20.87 v50.8,24.64
  pour Top (isolate 0.305, no thermals): 17.27,40.64 17.27,36.07 9.91,36.07 9.91,31.5 5.33,31.5 5.33,39.37 9.14,39.37 12.7,40.64
+INA
  Top 0.254: R47.2 15.66,20.23 14.73,19.3 14.73,16.76 14.99,16.51 15.76,16.51 U3.3 15.92,16.58 17.04,16.58 17.69,17.18 R45.2
+PVDD  (via drill 0.38 pad 0.64)
  Top 0.254: LED4.A 3.3,23.37 2.54,23.88 2.54,54.36 3.05,54.61 11.68,54.61 v11.94,54.86
  Top 1.27: Q3.7 20.57,49.58 21.59,48.51 27.05,40.13 C8.1 26.89,37.85 C9.1 | C2.1 C1.1 45.64,42.6 42.42,45.72 37.85,50.29 C29.1
  Bottom 0.254: R20.2 19.05,69.09 27.43,69.09 27.69,68.58 B+.1
  other vias: 18.29,55.88 19.3,55.88 20.57,55.88 21.59,55.88 18.29,54.86 18.29,53.85 18.29,52.83 19.3,54.86 19.3,53.85 19.3,52.83 20.57,54.86 20.57,53.85 20.57,52.83 21.59,54.86 21.59,53.85 21.59,52.83 53.34,52.83 54.36,52.83 53.34,53.85 54.36,53.85 54.36,54.86 53.34,54.86 53.34,55.88 54.36,55.88 35.56,52.83 36.58,52.83 35.56,53.85 36.58,53.85 36.58,54.86 35.56,54.86 35.56,55.88 36.58,55.88 37.85,52.83 38.86,52.83 37.85,53.85 38.86,53.85 38.86,54.86 37.85,54.86 37.85,55.88 38.86,55.88 55.63,52.83 56.64,52.83 55.63,53.85 56.64,53.85 56.64,54.86 55.63,54.86 55.63,55.88 56.64,55.88 13.46,60.71 13.46,58.67 13.46,56.9 13.46,54.86 13.46,53.09 11.94,60.71 11.94,58.67 11.94,56.9 11.94,53.09
  pour Top (isolate 0.305, rank 2, no thermals): 26.38,35.05 26.38,34.29 30.3,33.27 30.3,31.62 30.79,31.62 30.79,33.75 28.96,34.76 27.14,35.07
  pour Bottom (isolate 0.305, no thermals): 24.38,68.07 30.73,68.07 30.73,63.25 33.78,62.23 33.78,60.2 36.83,60.2 36.83,57.91 57.91,57.91 57.91,52.32 7.87,52.32 7.87,61.47 22.61,61.47 24.38,64.26
  pour Top (isolate 0.305, no thermals): 52.83,56.13 52.83,50.55 53.85,50.55 53.85,48.51 56.39,48.51 56.39,50.55 57.4,50.55 57.4,56.13
  pour Top (no thermals): 35.05,56.13 35.05,50.55 36.07,50.55 36.07,48.26 38.61,48.26 38.61,50.55 39.37,50.55 39.37,56.13
  pour Top (isolate 0.305, no thermals): 17.78,56.13 17.78,50.55 18.54,50.55 18.54,48.26 21.08,48.26 21.08,50.55 22.1,50.55 22.1,56.13
  pour Top (isolate 0.305, no thermals): 7.87,61.47 7.87,49.02 14.22,49.02 14.22,61.47
  pour Top (isolate 0.305, no thermals): 42.73,32.8 42.73,31.37 43.32,31.37 43.32,31.39 46.36,33.99 46.37,35.63 45.08,35.63 45.08,34.01 42.93,33.02
BIAS/VDD_SPI  (via drill 0.38 pad 0.64)
  Top 0.254: U1.49 32.83,32.07 32.83,33.11 32.77,33.36 32.26,34.69 31.32,35.88 v31.32,41.16
  Bottom 0.254: v31.32,41.16 23.11,41.15 | 23.11,41.15 C19.1 | R14.2 23.11,41.15
DC_CAL  (via drill 0.38 pad 0.64)
  Top 0.254: U1.12 34.82,24.09 34.82,16.76 34.04,16 34.04,12.45 | R9.1 33.11,10.76 34.04,11.68 34.04,12.45 | 34.04,12.45 v33.02,12.45 | U4.42 v57.91,35.31 | v44.7,12.45 46.23,10.92 66.8,10.92 66.8,34.8 66.04,35.31 66.04,37.08 60.96,37.08 v59.69,36.58
  Bottom 0.254: v44.7,12.45 v33.02,12.45 | v59.69,36.58 58.17,35.31 v57.91,35.31
DC_V_FB  (via drill 0.38 pad 0.64)
  Top 0.254: U4.6 51.56,28.7 50.55,29.72 48.26,29.72 47.24,30.73 47.24,31.5 | U2.I/O1 60.84,39.49 60.83,39.5 60.2,39.12 58.17,39.12 55.63,36.58 52.58,36.58 51.82,35.81 51.82,33.78 51.31,33.27 48.26,33.27 47.24,32.51 47.24,31.5 | 47.24,31.5 v46.23,31.5
  Bottom 0.254: C23.1 R22.2 R20.1 5.93,66.38 5.33,65.79 5.33,40.39 7.37,38.35 17.02,38.35 23.11,32.51 44.7,32.51 45.47,31.5 v46.23,31.5
DVDD  (via drill 0.38 pad 0.64)
  Top 0.254: U1.23 40.32,21.98 41.47,20.83 45.21,20.83 46.03,20.21 v46.03,19.95 | v47.5,27.69 48.1,27.69 C17.1
  Bottom 0.254: v46.03,19.95 45.97,27.69 v47.5,27.69
EN_GATE
  Top 0.254: R6.2 38.19,10.76 39.37,11.94 | 39.37,11.94 39.37,16.76 36.82,19.81 U1.16 | 39.37,11.94 40.39,10.16 67.56,10.16 67.56,25.91 68.58,25.91 69.09,26.42 69.09,37.08 68.58,37.59 58.93,37.59 58.42,37.08 58.42,36.32 58.93,35.81 58.93,34.8 58.42,34.29 U4.41
FAULT  (via drill 0.38 pad 0.64)
  Top 0.254: U1.6 31.83,24.05 31.83,21.8 29.97,19.69 29.97,13.97 v30.48,13.46 | Q2.1 24.83,7.3 25.15,7.87 25.15,10.5 R3.1 23.88,9.82 v23.88,9.4 | U4.48 54.91,33.83 v55.37,34.29 | v56.13,38.61 55.37,37.85 55.37,37.59 52.32,37.59 51.05,36.32 51.05,34.54 50.8,34.29 v49.02,34.29 | v23.11,34.29 v23.11,27.69
  Bottom 0.254: v30.48,13.46 30.48,11.94 29.21,10.67 29.21,8.89 28.7,8.38 24.38,8.38 v23.88,9.4 24.38,9.91 26.42,9.91 26.67,10.16 26.67,11.94 27.18,12.45 27.18,26.42 25.91,27.69 v23.11,27.69 | v55.37,34.29 55.37,37.85 v56.13,38.61 | v49.02,34.29 45.97,34.29 44.96,33.27 24.89,33.27 v23.11,34.29
GAIN/SDO  (via drill 0.38 pad 0.64)
  Top 0.254: U1.10 33.78,24.03 33.78,18.54 v33.27,18.29 | v64.52,26.19 U4.26
  Bottom 0.254: v33.27,18.29 32.77,17.78 32.77,14.73 45.97,14.73 48.26,12.45 65.02,12.45 65.02,14.22 64.26,14.99 60.2,14.99 58.67,16.26 58.67,22.86 59.44,22.86 62.23,25.4 62.23,25.93 62.75,26.19 v64.52,26.19
GH_A  (via drill 0.38 pad 0.64)
  Top 0.254: U1.47 33.82,33.54 33.78,33.78 33.27,35.31 32.77,36.07 v32.77,36.58 | v18.54,44.45 17.53,45.21 R28.1
  Bottom 0.254: v32.77,36.58 32.77,41.15 32.26,41.91 24.89,41.91 22.1,44.45 v18.54,44.45
GH_B  (via drill 0.38 pad 0.64)
  Top 0.254: U1.42 36.32,36.07 v36.07,36.58 | v35.56,42.42 34.04,43.94 R29.1
  Bottom 0.254: v36.07,36.58 36.07,41.91 v35.56,42.42
GH_C  (via drill 0.38 pad 0.64)
  Top 0.254: U1.37 38.82,36.16 v39.12,36.5 | v51.31,39.62 51.31,40.13 51.82,40.64 R30.1
  Bottom 0.254: v39.12,36.5 43.12,36.46 43.95,36.46 46.99,38.35 49.53,38.35 50.55,39.62 v51.31,39.62
GL_A
  Top 0.254: U1.45 34.82,33.9 34.82,34.11 34.15,36.07 34.14,40.42 31.24,43.94 R31.1
GL_B  (via drill 0.38 pad 0.64)
  Top 0.254: U1.40 37.32,34.17 v37.32,41.39 | v49.02,39.62 R32.1
  Bottom 0.254: v37.32,41.39 37.32,40.27 38.35,39.12 40.13,37.34 43.69,37.34 47.5,39.62 v49.02,39.62
GL_C  (via drill 0.38 pad 0.64)
  Top 0.254: U1.35 39.83,35.33 40.64,36.14 40.64,36.83 v40.64,38.35 | v67.04,42.16 67.04,42.4 67.31,42.67 67.31,45.96 R33.1
  Bottom 0.254: v40.64,38.35 43.69,38.35 47.5,40.64 58.67,40.64 59.18,40.13 65.28,40.13 65.53,40.39 v67.04,42.16
GND  (via drill 0.38 pad 0.64)
  Top 0.254: U1.30 42.32,33.72 44.2,34.94 | 44.19,34.95 arc45 44.2,34.94 | 44.2,34.94 v44.21,41.77 | C1.2 v47.16,36.86 | U1.32 41.32,34.23 41.32,34.45 43.07,35.73 43.07,39.62 41.52,42.4 41.49,42.48 v41.49,43.81 | U1.28 42.82,23.48 42.93,23.37 45.89,23.37 C16.2 46.39,25.15 | 46.39,25.15 46.39,25.4 | v44.7,24.89 45.47,25.4 46.39,25.4 | 46.39,25.4 C17.2 | C26.1 54.61,16.26 50.55,16.26 | 50.55,16.26 49.53,16.26 49.53,25.15 | 49.53,25.15 46.39,25.15 | C27.1 50.55,16.26 | 58.67,16 C25.1 | 63.75,40.13 63.5,40.39 60.96,40.39 v60.96,41.15 | U2.VN2 63.75,40.13 | 63.75,40.13 64.01,40.39 67.82,40.39 v68.07,40.13 | U4.12 50.09,25.7 | v49.53,26.42 49.53,25.91 49.89,25.91 50.09,25.7 | 49.53,25.15 50.09,25.7 | 53.85,33.53 53.85,34.54 54.61,35.05 56.39,35.05 56.9,34.54 U4.44 56.9,31.75 56.13,31.24 54.86,31.24 53.68,32.51 | R56.1 7.45,4.48 v7.37,4.57 | U4.30 60.96,28.19 v59.69,28.96
  Top 0.305: U4.30 63.5,28.19
  Top 0.406: 63.5,28.19 64.01,28.7 v64.26,28.7 v64.26,29.7
  Bottom 0.254: v44.21,41.77 45.58,42.9 arc45 45.59,42.93 45.97,42.93 48.77,42.93 50.33,42.92 50.33,44.4 C32.2 50.39,47.16 51.31,47.75 R35.1 | v41.49,43.81 34.15,43.8 C31.2 33.11,46.66 33.78,47.24 R34.1 | R36.1 65.86,46.94 C33.2 65.87,43.78 65.53,43.18 63.25,43.18 63.25,43.94 62.48,44.7 60.71,44.7 60.45,44.45 v59.44,44.45 | C36.2 53.68,33.53 C35.2 C34.2 | C40.2 66.29,32.6 66.29,32 65.44,31.15 C42.2 65.42,29.7 v64.26,29.7
  Bottom 0.508: 53.85,33.53 53.68,33.53
  other vias: 30.99,26.92 30.99,28.07 30.99,29.21 32.26,26.92 32.26,28.07 32.26,29.21 33.53,26.92 33.53,28.07 33.53,29.21 34.8,26.92 34.8,28.07 34.8,29.21 36.07,26.92 36.07,28.07 36.07,29.21 37.34,26.92 37.34,28.07 37.34,29.21 38.61,26.92 38.61,28.07 38.61,29.21 39.88,26.92 39.88,28.07 39.88,29.21 41.15,26.92 41.15,28.07 41.66,29.21 44.96,26.42 17.02,65.79 15.49,64.77 15.49,62.74 17.53,62.74 20.07,62.74 23.11,65.79 11.94,62.74 8.89,62.74 22.35,63.75 15.24,8.64 16.76,8.64 18.29,8.64 35.56,9.65 36.07,8.38 39.37,7.37 10.16,23.62 11.68,28.7 17.27,28.7 18.29,21.08 9.14,28.7 36.58,11.68 42.67,11.68 35.81,44.45 37.08,44.45 38.35,44.45 19.05,40.89 20.83,41.15 53.59,43.69 52.83,44.96 54.61,44.96 55.88,44.96 54.61,20.57 55.63,16 7.11,46.48 7.11,44.96 9.65,44.96 9.65,46.48 12.7,46.48 12.7,44.96 55.63,30.23 53.59,33.53 71.37,38.1 71.37,34.04 71.37,30.73 71.37,27.69 71.37,25.4 65.28,23.11 57.91,14.99 58.67,14.22 70.61,68.33 67.56,68.33 64.77,68.33 64.77,66.29 67.56,66.29 70.61,67.06 70.61,65.53 70.61,64.01 70.61,62.23 68.33,62.23 67.56,64.26 65.79,64.26 32.77,68.83 40.13,68.83 42.16,68.83 41.66,67.31 2.29,68.07 6.6,68.33 10.92,68.33 2.29,62.48 2.29,57.66 2.29,20.07
  pour Top (isolate 0.305, no thermals): 7.37,41.4 10.41,41.4 10.41,45.97 7.37,45.97
  pour Top (no thermals): 7.37,63.75 10.41,63.75 10.41,68.33 7.37,68.33
  pour Top (no thermals): 61.21,30.23 64.77,30.23 65.02,29.97 65.02,29.46 64.77,29.21 64.26,29.21 64.01,29.46 64.01,29.72 61.21,29.72
  pour Top (isolate 0.305, no thermals): 64.26,33.27 64.26,32.51 64.77,32.51 64.77,30.48 64.01,29.72 64.01,29.46 64.26,29.21 64.77,29.21 65.53,29.97 65.53,33.02 65.28,33.27
  pour Bottom (isolate 0.305, no thermals): 51.05,45.97 51.31,45.72 53.34,45.72 53.59,45.97 53.59,49.78 53.34,50.04 51.05,50.04
  pour Bottom (isolate 0.305, no thermals): 66.55,49.28 68.83,49.28 68.83,45.97 68.33,45.47 66.55,45.47 66.29,45.72 66.29,49.02
  pour Bottom (isolate 0.305, rank 6): 1.02,68.58 1.02,2.29 2.29,1.02 71.37,1.02 72.14,1.78 72.14,68.83 71.37,69.6 2.03,69.6
  pour Top (isolate 0.305, rank 6): 2.03,69.6 1.02,68.58 1.02,2.29 2.29,1.02 71.37,1.02 72.14,1.78 72.14,68.83 71.37,69.6
GPIO33
  Top 0.254: 61.72,31.24 62.23,31.24 | 62.23,31.24 62.99,31.24 | U4.36 62.23,31.24
  pour Top (isolate 0.254, no thermals): 62.23,31.75 63.25,32 63.24,31.2 62.22,31.2
GPIO34  (via drill 0.38 pad 0.64)
  Top 0.254: U4.19 57.91,25.15 56.9,25.91 56.9,28.19 v57.66,29.97 | v69.6,22.35 69.09,22.35 69.09,9.65 69.85,8.89 69.85,3.56 69.6,3.3 3.81,3.3 3.3,3.81 3.3,10.92 JP1.2
  Top 0.406: R55.2 JP1.2
  Bottom 0.254: v57.66,29.97 58.17,30.48 58.17,34.04 56.9,34.8 56.9,35.81 59.44,37.85 69.09,37.85 69.6,37.34 69.6,30.48 68.07,30.48 67.82,30.23 67.82,28.96 67.31,28.45 66.29,28.45 66.29,24.38 67.06,24.38 68.83,22.86 69.09,22.35 v69.6,22.35
IA_FB
  Top 0.203: 52.58,18.03 57.66,18.03
  Top 0.254: R25.1 52.58,18.03 | 57.66,18.03 57.66,16 56.39,14.73 49.02,14.73 48.01,15.75 48.01,21.34 47.5,21.84 41.91,21.84 41.32,22.44 U1.25 | U1.25
IB_FB
  Top 0.254: U1.26 41.82,22.7 42.16,22.35 48.01,22.35 48.77,21.59 48.77,16 49.53,15.24 56.13,15.24 56.64,15.75 R26.1
IC_FB  (via drill 0.38 pad 0.64)
  Top 0.254: U3.1 15.83,14.14 16,13.72 16,13.3 R43.2 v17.53,13.21 | v62.23,17.53 61.3,17.53 R27.1
  Bottom 0.254: v17.53,13.21 17.53,11.18 25.4,3.3 52.07,3.3 53.34,2.03 65.28,2.03 67.56,4.32 67.56,6.1 70.36,6.1 70.36,17.78 64.52,22.61 62.48,22.61 60.96,21.08 60.96,17.53 v62.23,17.53
M_OC/SDI  (via drill 0.38 pad 0.64)
  Top 0.254: U1.9 33.32,19.98 v32.77,19.56 | v64.52,27.43 63.78,26.7 U4.27
  Bottom 0.254: v32.77,19.56 31.75,19.56 31.75,10.67 66.55,10.67 66.55,15.24 65.28,16.51 60.96,16.51 60.2,17.02 60.2,21.59 62.74,23.88 63.25,24.38 64.01,24.38 64.26,24.13 65.53,24.13 65.53,27.18 65.28,27.43 v64.52,27.43
M_PWM/SCS  (via drill 0.38 pad 0.64)
  Top 0.254: U4.25 61.93,25.65 62.74,25.65 63.25,25.15 v64.52,25.15 | v33.02,13.72 33.02,13.95 32.01,14.95 32,16.51 32,19.05 31.75,19.3 31.75,19.85 32.82,20.92 32.82,22.08 U1.8
  Bottom 0.254: v33.02,13.72 45.21,13.72 47.5,11.43 65.79,11.43 65.79,14.73 64.77,15.75 60.45,15.75 59.44,16.51 59.44,21.84 62.99,25.15 v64.52,25.15
N$1
  Top 0.254: U1.4 | U1.4 30.82,22.57 29.84,21.59 28.7,21.59 28.45,21.34 R10.1
N$2
  Top 0.254: U1.3 30.32,22.86 29.55,22.1 27.43,22.1 26.92,21.59 26.92,19.56 26.42,18.54 R7.2 R8.1
N$3
  Top 0.254: U1.52 31.31,33.75 31.31,33.96 30.19,35.21 30.19,36.77 | 30.05,37.05 30.19,36.77 | 30.19,36.77 C10.2
N$4
  Top 0.254: U1.7 32.34,24.07 32.34,21.43 30.99,19.91 R5.2
N$5  (via drill 0.38 pad 0.64)
  Top 0.254: 31.82,33.34 U1.51 | U1.50 32.33,32.07 32.33,32.83 31.82,33.34 | 31.82,33.34 31.82,34.22 31.75,34.29 30.77,35.41 30.77,35.88 30.77,38.4 29.97,38.93 C10.1 29.72,39
  Top 0.508: v21.08,37.85 21.08,35.56 17.02,33.27 15.24,33.27 L1.2 15.24,27.6 D3.C | v29.72,40.13 29.72,39
  Bottom 0.508: v29.72,40.13 24.13,40.13 22.86,37.85 v21.08,37.85
N$6
  Top 0.254: R12.2 C18.1
N$7
  Top 0.254: U1.56 26.88,32.07 C14.1
N$8
  Top 0.254: Q1.3 30.72,5.35 LED1.A
N$9
  Top 0.254: U1.2 29.82,23.17 29.51,22.86 26.42,22.86 25.65,22.1 R12.1 25.49,22.1 24.89,22.1 24.64,22.35 24.64,23.11 23.88,23.11 23.88,23.88 23.71,24.04 C15.1
N$10
  Top 0.254: U1.15 36.32,19.3 38.1,17.02 C3.1
N$11
  Top 0.254: U1.1 29.29,24.04 R11.1
N$12
  Top 0.254: C3.2 36.83,14.9 36.83,17.53 35.82,18.77 U1.14
N$13
  Top 0.254: C4.1 35.32,14.67 U1.13
N$14
  Top 0.254: U1.43 35.81,35.07 35.31,36.07 35.31,37.08 35.81,37.59 C6.1
N$15
  Top 0.254: U1.48 33.33,33.32 33.27,33.53 32.77,35.05 32,36.07 32,37.59 C5.1
N$16
  Top 0.254: U1.38 38.32,36.78 38.87,37.53 C7.1
N$17
  Top 0.254: LED1.C 33.4,5.71 34.04,5.08 36.74,5.08 R1.1
N$18
  Top 0.254: LED2.A 24.05,5.43 Q2.3
N$19
  Top 0.254: LED2.C 17.58,7.53 R4.1
N$20  (via drill 0.38 pad 0.64)
  other vias: 59.44,56.13
N$21
  Top 0.254: R47.1 15.07,21.93 14.48,21.34 14.48,20.57 14.22,20.32 13.3,20.32 C38.1 13.21,20.07 13.97,19.3 13.97,16.76 13.72,16.51 13.2,16.51 U3.6 U3.7
N$22
  Top 0.254: R46.1 R48.2 13.08,17.18 U3.5
N$23
  Top 0.254: U1.27 42.32,22.96 42.42,22.86 47.75,22.86 48.09,23.2 C16.1
N$24
  Top 0.254: R28.2 16.26,56.39 17.02,57.45 Q3.4
N$25
  Top 0.254: R29.2 34.04,56.9 34.54,57.4 34.56,57.45 Q4.4
N$26
  Top 0.254: R43.1 14.48,13.3 14.48,15.75 14.66,15.93 U3.2 15.91,15.93 16.78,15.93 17.53,15.24 R44.2
N$27
  Top 0.254: Q5.4 52.07,57.45 51.82,56.9 R30.2
N$28
  Top 0.254: Q7.4 47.98,50.5 49.02,49.78 R32.2
N$29
  Top 0.254: Q8.4 65.28,50.8 67.27,49.55 R33.2
N$30
  Top 0.254: Q6.4 30.46,50.03 31.24,49.53 R31.2
N$31
  Top 0.254: U4.15 55.91,20.55 56.64,19.81 R26.2 C26.2
N$32
  Top 0.254: C27.2 R25.2 52.58,20.32 54.48,22.1 54.91,22.53 54.91,23.11 U4.13
N$33
  Top 0.254: R50.2 41.4,7.15 LED3.C
N$34
  Top 0.254: LED4.C 6.6,23.15 6.6,22.35 7.02,22.01 R23.2
N$35
  Top 0.254: C25.2 R27.2 60.71,19.81 58.42,19.81 57.4,20.83 U4.18
N$36
  Top 0.254: LED5.C 15.17,5.55 R24.2
N$37  (via drill 0.38 pad 0.64)
  other vias: 59.44,54.86
N$38  (via drill 0.38 pad 0.64)
  other vias: 58.42,43.43
N$39
  Top 0.254: R54.2 47.5,6.1 JTAG.13
N$40
  Top 0.254: R53.2 JTAG.14
N$42
  Top 0.254: R57.2 JP1.1
N$44
  Bottom 0.254: R21.1 35.71,61.98 38.1,61.98 38.77,61.3 C24.1
N$45
  Top 0.406: JP2.1 R58.2
OC_ADJ/SCLK  (via drill 0.38 pad 0.64)
  Top 0.254: v33.78,17.02 34.32,17.55 U1.11
  Bottom 0.254: R16.1 33.78,15.49 v33.78,17.02
OCTW  (via drill 0.38 pad 0.64)
  Top 0.254: U1.5 31.33,22.12 29.47,20.01 29.46,13.97 v29.21,13.46 | v27.94,9.4 27.94,10.07 R2.1 28.79,10.83 29.21,10.16 29.21,7.62 Q1.1 | U4.1 49.48,31.19 v49.02,31.5
  Bottom 0.254: v27.94,9.4 27.94,12.45 28.19,12.7 28.7,12.7 v29.21,13.46 29.49,13.75 29.49,20.04 31.24,22.04 31.24,22.1 42.67,22.1 43.43,22.86 43.43,28.7 43.94,29.21 46.48,29.21 v49.02,31.5
PWM_AH  (via drill 0.38 pad 0.64)
  Top 0.254: U1.17 37.34,24.05 37.34,20.07 40.89,16.26 v43.18,16.26 | U4.29 60.2,27.69 59.69,27.94 v58.93,27.94
  Bottom 0.254: v58.93,27.94 59.94,27.94 59.94,26.16 58.67,25.15 54.86,25.15 47.24,16.26 v43.18,16.26
PWM_AL  (via drill 0.38 pad 0.64)
  Top 0.254: U1.18 37.82,20.47 40.89,17.27 v41.91,17.27 | v58.93,26.67 59.69,26.67 60.22,27.2 U4.28
  Bottom 0.254: v41.91,17.27 46.99,17.27 54.36,25.91 57.91,25.91 v58.93,26.67
PWM_BH
  Top 0.254: U1.19 38.32,20.86 40.89,18.29 42.93,18.29 44.7,16.51 44.7,14.73 47.5,11.68 66.29,11.68 66.29,34.04 62.48,34.04 61.98,33.53 60.45,33.53 | 60.45,32.72 U4.37
  Top 0.305: 60.45,33.53 60.45,32.72
PWM_BL  (via drill 0.38 pad 0.64)
  Top 0.254: U1.20 38.82,21.13 40.89,19.05 43.18,19.05 45.47,16.76 45.47,15.24 48.01,12.45 63.75,12.45 v63.75,13.46 | U4.38 59.94,32.69 59.94,33.78 60.45,34.29 61.98,34.29 v62.23,35.05
  Bottom 0.254: v63.75,13.46 62.99,14.22 59.94,14.22 57.91,16 57.91,23.62 59.18,23.62 61.47,25.65 61.47,33.27 62.23,34.04 v62.23,35.05
PWM_CH  (via drill 0.38 pad 0.64)
  Top 0.254: U1.21 39.32,21.39 40.95,19.76 43.49,19.76 46.23,17.02 46.23,15.49 48.26,13.46 v52.83,13.46 | U4.39 59.44,32.69 59.44,34.04 60.2,34.8 60.71,34.8 v62.23,36.32
  Bottom 0.254: v62.23,36.32 60.71,34.8 60.71,25.91 58.93,24.38 55.12,24.38 52.83,21.59 v52.83,13.46
PWM_CL
  Top 0.254: U1.22 39.82,21.65 41.15,20.32 43.94,20.32 46.99,17.27 46.99,15.75 48.51,14.22 53.34,14.22 54.86,12.95 61.72,12.95 62.23,13.46 62.23,13.97 62.74,14.48 64.77,14.48 65.28,14.99 65.28,21.84 62.74,24.13 61.72,24.13 61.47,24.64 60.45,25.65 58.67,25.65 57.66,26.42 57.66,28.45 58.93,29.97 58.93,32.64 U4.40
RESET#
  Top 0.254: R49.1 51.7,22.49 55.12,25.91 56.13,25.91 56.13,27.69 55.63,28.19 54.86,28.19 54.86,29.72 54.61,30.23 53.47,30.23 U4.3
SCLK  (via drill 0.38 pad 0.64)
  Top 0.254: U4.24 60.4,23.67 60.45,23.62 62.48,23.62 64.52,21.84 64.52,15.49 64.26,15.24 62.48,15.24 60.71,13.46 56.13,13.46 v55.88,13.97
  Bottom 0.254: R16.2 54.36,15.49 54.61,15.24 55.05,14.99 55.63,14.73 v55.88,13.97
SH_A
  Top 0.254: U1.46 34.32,33.51 34.29,33.78 33.53,36.32 33.53,38.35 C5.2 32.39,41.52 31.5,42.67 27.43,42.67 23.11,49.53 23.11,52.32 Q6.9
  Bottom 0.254: R37.1 41.49,64.26 39.88,64.26 39.88,65.79 A.1
  pour Top (isolate 0.305, no thermals): 36.58,68.33 38.35,68.33 39.88,67.06 39.88,64.52 33.78,58.42 30.99,58.42 30.99,53.09 26.16,53.09 26.16,56.13 25.15,57.15 19.05,57.15 19.05,58.67 29.97,62.23
SH_B  (via drill 0.38 pad 0.64)
  Top 0.254: U1.41 36.83,38.86 C6.2 35.81,40.39 35.91,40.65 36.93,42.68 38.66,42.68 v40.13,45.21 | v41.15,50.8 41.15,52.83 Q7.9
  Bottom 0.254: v40.13,45.21 41.15,46.74 v41.15,50.8 | R39.1 51.56,63.25 B.1
  pour Top (isolate 0.305, no thermals): 45.72,68.33 48.01,68.33 49.28,67.31 49.28,63.25 48.51,61.72 48.51,53.09 43.69,53.09 43.69,57.15 36.32,57.15 36.32,58.17
SH_C  (via drill 0.38 pad 0.64)
  Top 0.254: U1.36 39.32,35.2 39.32,35.52 40.08,36.37 40.08,37.63 39.82,38.14 39.82,39.97 | 39.82,39.97 C7.2 | 39.82,39.97 v40.56,39.96 | 61.98,54.61 62.74,54.61 | 62.74,54.61 62.94,54.61 Q8.9 | 62.74,54.61 59.18,53.59 59.18,51.05 57.91,49.28 57.15,49.02 57.15,44.96 55.37,43.18 v55.37,42.93
  Bottom 0.254: v40.56,39.96 40.89,40.39 44.2,40.39 46.74,42.16 55.12,42.16 v55.37,42.93 | R41.1 60.45,61.72 C.1
  pour Top (isolate 0.305, no thermals): 53.85,68.33 53.85,64.26 54.1,63.5 54.1,57.15 59.94,57.15 60.71,56.39 60.71,53.34 60.96,53.09 65.79,53.09 65.79,58.42 57.91,68.33
SL_A  (via drill 0.38 pad 0.64)
  Top 0.254: U1.33 40.82,32.93 40.83,34.78 42.53,36.2 42.53,38.92 42.53,39.34 42.51,39.37 41.66,40.64 v40.39,42.67 | U1.44 35.32,34.79 34.8,35.81 34.8,40.64 v34.29,41.66
  Bottom 0.254: v40.39,42.67 39.89,43.26 33.44,43.26 31.44,43.26 | 31.44,43.26 31.4,43.26 31.41,43.43 C31.1 | v34.29,41.66 32.77,42.67 29.46,42.67 R34.2 30.73,47.24 31.41,46.51 31.41,44.24 31.41,43.27 31.44,43.26
  other vias: 27.18,46.99 26.42,48.01 25.65,49.02 27.18,49.02 26.67,50.04 25.15,50.04
  pour Top (isolate 0.305, no thermals): 29.46,52.07 29.46,45.97 26.92,45.97 24.13,50.29 24.13,52.07
  pour Bottom (isolate 0.305, no thermals): 24.13,50.55 30.48,50.55 30.48,45.97 26.92,45.97 24.13,50.29
SL_B  (via drill 0.38 pad 0.64)
  Top 0.254: U1.39 37.82,37.35 37.82,37.59 37.82,40.59 38.35,41.15 v39.12,41.4 | U1.31 41.84,33.82 41.84,34.05 43.62,35.34 43.61,40.5 v42.82,41.96
  Bottom 0.254: v39.12,41.4 40.89,41.4 45.97,46.48 45.97,48.51 R35.2 47.5,47.5 47.65,47.45 48.68,46.93 C32.1 45.47,44.45 v42.82,41.96
  other vias: 43.69,49.28 43.69,50.29 44.7,49.78 44.7,48.77 44.7,47.75 43.69,48.26
  pour Top (isolate 0.305, no thermals): 43.69,52.07 46.99,52.07 46.99,46.48 43.94,46.48 43.18,47.24 43.18,51.05
  pour Bottom (isolate 0.305, no thermals): 43.43,51.31 45.97,51.31 47.24,50.55 47.75,50.55 47.75,45.97 43.18,45.97 43.18,51.05
SL_C  (via drill 0.38 pad 0.64)
  Top 0.254: U1.34 40.33,35.07 41.65,36.23 41.67,36.54 41.66,37.07 v41.67,39.11 | R44.1 20.57,15.24 v20.83,14.99 | v69.09,43.94 70.36,42.42 70.36,25.91 69.09,24.64 69.09,23.37 70.1,23.37 70.61,22.86 70.61,21.84 69.85,21.08 69.85,10.16 70.61,9.4 70.61,2.79 70.36,2.54 3.3,2.54 2.54,3.3 2.54,16 3.3,16.76 v4.32,16.76
  Bottom 0.254: v41.67,39.11 43.43,39.12 46.99,41.4 55.63,41.4 56.39,42.16 56.39,43.43 v58.93,45.97 | R36.2 64.18,46.97 C33.1 64.17,48.68 65.28,49.78 65.28,50.29 69.6,50.29 69.6,44.7 v69.09,43.94 | v20.83,14.99 20.57,15.24 4.32,15.24 v4.32,16.76
  other vias: 58.93,46.99 59.94,46.99 58.93,48.01 59.94,48.01 59.94,49.02
  pour Top (isolate 0.305, no thermals): 60.45,52.07 64.26,52.07 64.26,45.47 58.42,45.47 58.42,48.01 60.45,50.55
  pour Bottom (isolate 0.305, no thermals): 62.99,49.78 59.94,49.78 59.82,49.77 58.42,48.01 58.42,45.47 62.99,45.47
TCK  (via drill 0.38 pad 0.64)
  Top 0.254: U4.23 59.92,23.14 60.2,22.86 61.98,22.86 v63.5,21.34 | JTAG.9 JTAG.11
  Bottom 0.254: JTAG.9 52.83,3.56 53.59,2.79 64.77,2.79 66.8,4.83 66.8,6.86 69.38,6.86 69.62,6.85 69.62,17.34 64.52,21.59 v63.5,21.34
TDI  (via drill 0.38 pad 0.64)
  Top 0.254: U4.20 58.42,21.34 58.93,20.57 60.96,20.57 v62.23,18.8
  Bottom 0.254: v62.23,18.8 62.48,19.05 65.02,19.05 68.07,16.26 68.07,8.38 65.28,8.38 65.28,5.33 64.01,4.06 60.96,4.06 60.45,4.57 JTAG.3
TDO  (via drill 0.38 pad 0.64)
  Top 0.254: U4.22 59.41,22.63 59.94,22.1 61.47,22.1 v63.5,20.07 | JTAG.7 55.37,4.57 54.86,4.06 10.92,4.06 10.76,4.23 10.76,5.75 10.41,6.1 9.23,6.1 R56.2 JP2.2
  Bottom 0.254: v63.5,20.07 64.77,20.32 68.83,16.76 68.83,7.62 66.04,7.62 66.04,5.08 64.52,3.56 55.88,3.56 55.37,4.32 JTAG.7
TMS  (via drill 0.38 pad 0.64)
  Top 0.254: U4.21 58.9,22.12 59.69,21.34 61.21,21.34 63.5,18.8 v63.5,18.03
  Bottom 0.254: JTAG.1 64.52,5.84 64.52,9.14 67.31,9.14 67.31,15.75 64.77,18.03 v63.5,18.03
TRST
  Top 0.254: U4.2 49.51,30.71 49.28,30.48 48.51,30.48 48.01,30.99 48.01,32 48.77,32.51 51.56,32.51 52.58,33.53 52.58,35.31 52.83,35.81 55.88,35.81 58.42,38.35 69.34,38.35 69.85,37.85 69.85,26.16 69.09,25.4 68.33,25.4 68.33,9.4 63.5,9.4 63.5,8.89 JTAG.2
  Top 0.406: JTAG.2 65.53,8.38 R51.2
VA_FB  (via drill 0.38 pad 0.64)
  Top 0.254: U4.7 51.31,28.19 50.55,28.7 v49.53,28.7 | v66.8,39.62 66.29,39.37 64.58,39.37 U2.I/O3
  Bottom 0.254: C34.1 50.8,36.83 50.04,36.07 50.04,28.7 v49.53,28.7 | C34.1 51.73,37.25 | R37.2 R38.2 | R37.2 42.76,59.6 42.67,59.69 | R37.2 45.63,59.6 45.72,59.69 45.72,61.98 43.18,64.77 43.18,67.06 45.21,69.09 58.93,69.09 68.33,58.17 68.33,53.85 71.12,51.31 71.12,42.16 68.33,42.16 68.07,41.91 66.8,40.39 v66.8,39.62 66.29,39.37 57.91,39.37 57.66,39.88 52.58,39.88 52.32,39.12 51.82,38.86 51.82,37.34 C34.1
VB_FB  (via drill 0.38 pad 0.64)
  Top 0.254: U4.8 v50.55,27.69 | U2.I/O4 64.7,42.74 64.52,43.18 61.72,43.18 | 61.72,43.18 59.94,43.18 59.44,42.67 59.44,40.64 58.93,40.13 56.13,40.13 v54.36,38.86 | v61.72,43.94 61.72,43.18
  Bottom 0.254: v54.36,38.86 54.36,38.61 52.58,37.85 52.58,35.56 51.47,34.71 C35.1 50.55,34.8 50.55,28.19 50.8,27.69 v50.55,27.69 | v61.72,43.94 61.72,42.42 66.04,42.42 66.55,43.18 67.56,43.18 67.82,42.93 70.36,42.93 70.36,50.8 67.56,53.34 67.56,57.91 66.55,58.93 62.48,58.93 61.72,59.69 61.72,60.45 53.59,60.45 52.74,59.6 R39.2 R40.2
VC_FB  (via drill 0.38 pad 0.64)
  Top 0.254: U4.10 53.43,26.71 v51.41,26.71 | U2.I/O6 62.8,41.08 62.99,40.89 67.31,40.89 67.56,41.15 68.33,41.15 | v67.56,51.56 68.58,50.29 68.58,44.96 68.07,44.45 68.07,43.43 68.33,43.18 68.33,41.15 | v69.09,41.15 68.33,41.15
  Bottom 0.254: v51.41,26.71 51.73,27.03 C36.1 52.07,32.51 52.07,30.99 55.63,30.99 57.4,32.77 57.4,33.53 56.13,34.54 56.13,36.32 58.93,38.61 69.09,38.61 v69.09,41.15 | v67.56,51.56 66.8,52.07 66.8,57.66 66.29,58.17 61.89,58.17 R41.2 R42.2
VDD1
  Top 0.254: C41.1 62.23,33.02 60.45,31.24 60.45,29.21 U4.32
VDD2  (via drill 0.38 pad 0.64)
  Top 0.254: U4.43 57.4,30.99 56.64,30.99 56.64,29.46 v56.39,29.21
  Bottom 0.254: v56.39,29.21 54.1,29.21 53.59,28.96 53.59,26.16 46.74,18.29 44.36,18.29 C39.1
VDDA  (via drill 0.38 pad 0.64)
  Top 0.254: U4.11 54.38,26.19 v55.12,27.18
  Bottom 0.254: v55.12,27.18 57.66,27.18 57.66,28.45 58.93,29.97 58.93,34.04 60.71,35.81 60.71,37.08 68.58,37.08 68.58,34.29 | 68.58,34.29 L2.2 | C42.1 66.64,31.15 68.58,32 68.58,34.29
VDDIO  (via drill 0.38 pad 0.64)
  Top 0.254: U4.35 63.78,30.71 v64.52,31.5
  Bottom 0.254: v64.52,31.5 64.26,31.75 64.26,32.77 | 64.26,32.77 64.26,33.02 63.25,34.04 63.25,35.05 64.26,36.07 L3.2 | C40.1 64.26,32.77

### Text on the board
tNames: PVDD | BOOT | BOOT | OCTW | JTAG | P.FISHER FOC ESC-REV 1 | FAULT | 3.3V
